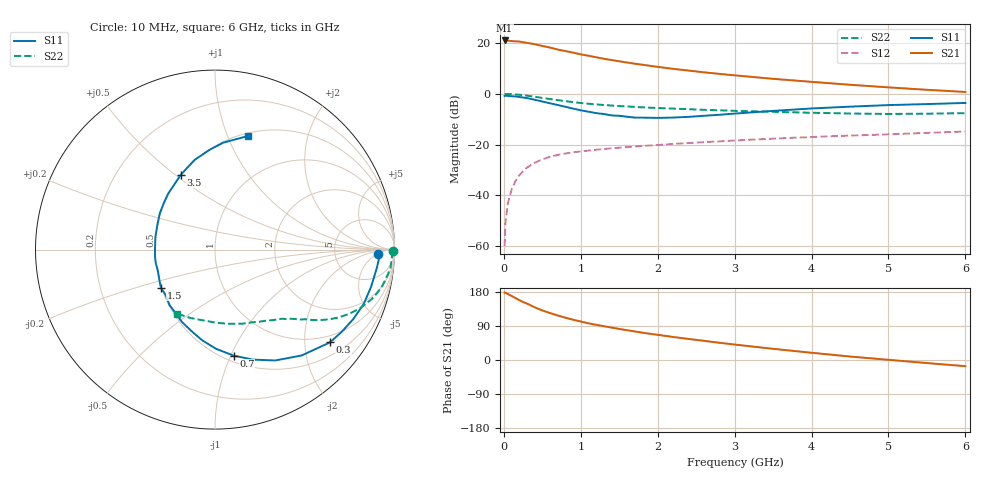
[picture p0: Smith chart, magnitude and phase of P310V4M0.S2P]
! SIEMENS Small Signal Semiconductors
! BFP181
! Si NPN RF Bipolar Junction Transistor in SOT143
! VCE = 10 V  IC = 4 mA
! Common Emitter S-Parameters:  March  1996
# GHz  S  MA  R  50
!  f  S11  S21  S12  S22
! GHz  MAG  ANG  MAG  ANG  MAG  ANG  MAG  ANG
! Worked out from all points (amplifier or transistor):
!   36 points, 10 MHz to 6 GHz, reference 50 ohm
!   highest |S21| = 21.0 dB at 10 MHz (marker M1)
!   |S21| within 3 dB of that: start of sweep to 625.2 MHz
!   unconditionally stable (mu >= 1): 2.05 GHz to end of sweep
!   at 250 MHz: K = 0.18, MSG = 25.4 dB, |S12| = -30.5 dB
!   at 1.4 GHz: K = 0.81, MSG = 17.4 dB, |S12| = -21.5 dB
!   at 6 GHz: K = 1.10, MAG = 5.9 dB, |S12| = -14.9 dB
!   S11 on the Smith chart (normalised r, x): 10 MHz: 19, -5; 300 MHz: 0.81, -2.61; 700 MHz: 0.56, -1.03; 1.5 GHz: 0.50, -0.24; 3.5 GHz: 0.50, +0.53; 6 GHz: 0.53, +1.19
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0.01  0.9078 -1.4  11.18 178.1  0.001 80.3  0.9904 -0.5
0.02  0.9164 -2.6  11.06 177.6  0.0028 76.8  0.9884 -1.2
0.05  0.9074 -6.5  11.05 174.3  0.0067 87.3  0.9856 -3.2
0.1  0.8939 -13.4  10.88 169.0  0.0129 79.9  0.9826 -6.3
0.2  0.8625 -26.6  10.64 158.2  0.0247 74.5  0.9542 -12.2
0.25  0.8419 -32.9  10.32 153.1  0.0298 71.4  0.9355 -15.0
0.3  0.8232 -38.9  10.03 148.9  0.0351 68.3  0.9162 -17.5
0.4  0.7622 -50.7  9.441 139.1  0.0438 62.7  0.8732 -21.9
0.5  0.7029 -61.5  8.723 130.8  0.051 57.3  0.8275 -25.7
0.6  0.6482 -71.0  8.092 123.9  0.0575 53.5  0.785 -28.8
0.7  0.5998 -80.0  7.402 117.6  0.0624 50.0  0.7476 -31.3
0.9  0.5106 -98.0  6.438 106.3  0.0705 44.9  0.6844 -35.0
1.1  0.4429 -114.6  5.595 96.8  0.0762 41.8  0.635 -37.7
1.3  0.399 -129.5  4.875 89.2  0.0817 39.2  0.6001 -40.2
1.5  0.3683 -145.0  4.358 82.0  0.0866 37.5  0.5727 -42.3
1.8  0.3385 -167.2  3.72 72.1  0.0934 35.7  0.5401 -45.5
2.2  0.3398 167.7  3.089 60.8  0.1027 33.3  0.51 -50.3
2.8  0.3851 138.0  2.46 45.5  0.1155 30.3  0.4721 -58.3
3.5  0.4593 114.4  1.966 29.5  0.1306 26.4  0.4407 -69.4
4.5  0.5567 93.1  1.501 9.2  0.15 20.3  0.408 -88.8
5.5  0.6256 79.3  1.195 -8.1  0.1698 15.2  0.4048 -109.7
6  0.659 73.8  1.083 -16.3  0.1804 11.9  0.4144 -120.6
